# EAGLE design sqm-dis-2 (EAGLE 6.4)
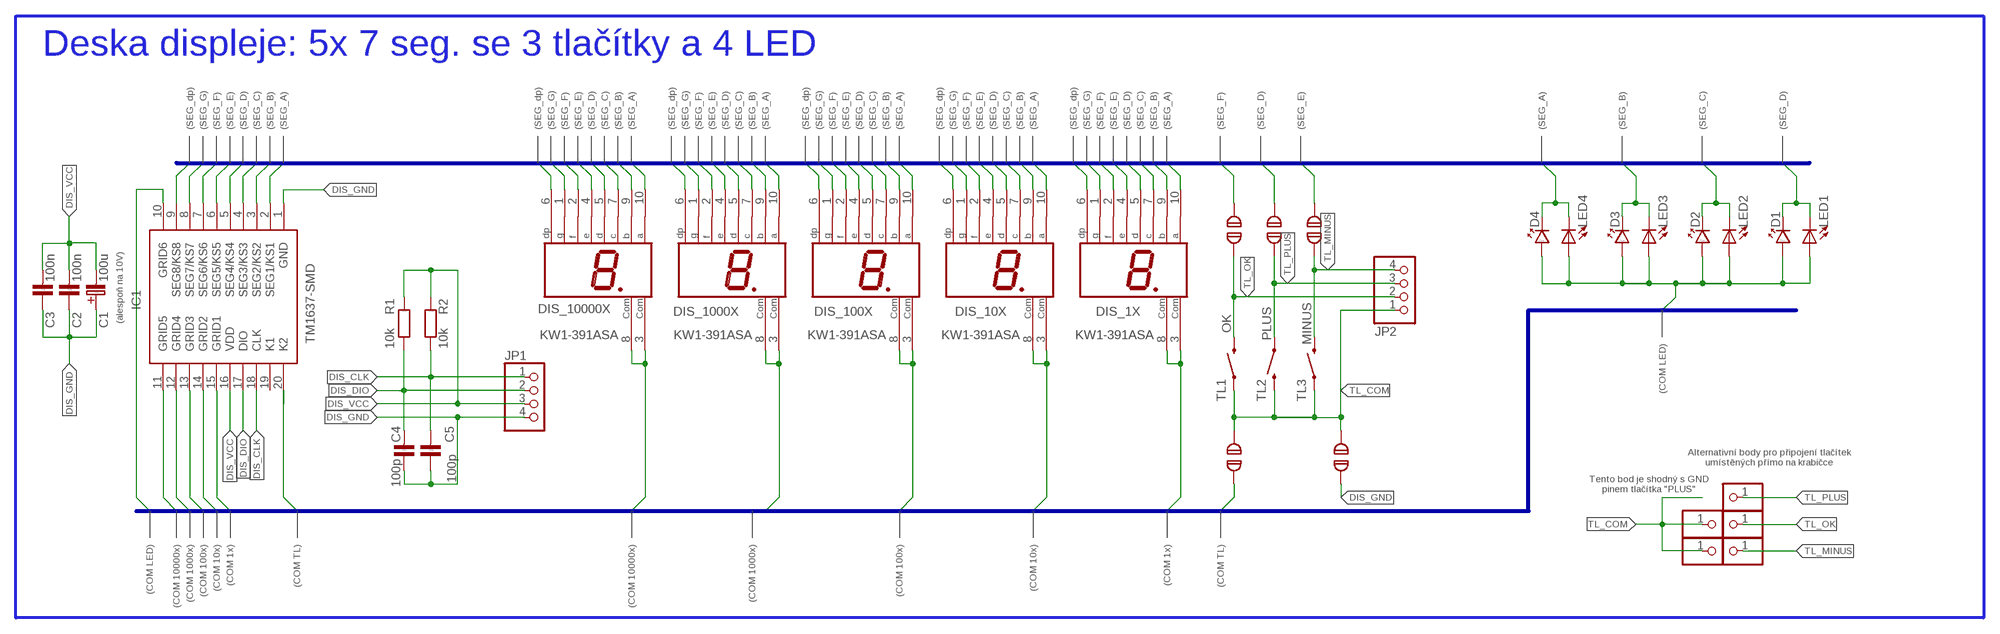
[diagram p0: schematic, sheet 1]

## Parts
C1  100u  C-ELEKTROLYT_2,5  [C-EL_2,5]
C2  100n  C-KERAMIK_SMD_0805  [0805]
C3  100n  C-KERAMIK_SMD_0805  [0805]
C4  100p  C-KERAMIK_SMD_0805  [0805]
C5  100p  C-KERAMIK_SMD_0805  [0805]
D1  LED_3  [LED_3]
D2  LED_3  [LED_3]
D3  LED_3  [LED_3]
D4  LED_3  [LED_3]
DIS_1X  KW1-391ASA  SC39-11SRWA  [HDSP-E]
DIS_10X  KW1-391ASA  SC39-11SRWA  [HDSP-E]
DIS_100X  KW1-391ASA  SC39-11SRWA  [HDSP-E]
DIS_1000X  KW1-391ASA  SC39-11SRWA  [HDSP-E]
DIS_10000X  KW1-391ASA  SC39-11SRWA  [HDSP-E]
IC1  TM1637-SMD  TM1637__SOP_  [SOIC127P1045X280-20N]
JP1  PINHD-1X4  [1X04]
JP2  PINHD-1X4  [1X04]
JP4  PINHD-1X1  [1X01]
JP5  PINHD-1X1  [1X01]
JP6  PINHD-1X1  [1X01]
JP7  PINHD-1X1  [1X01]
JP8  PINHD-1X1  [1X01]
LED1  LEDCHIP-LED0805  [CHIP-LED0805]
LED2  LEDCHIP-LED0805  [CHIP-LED0805]
LED3  LEDCHIP-LED0805  [CHIP-LED0805]
LED4  LEDCHIP-LED0805  [CHIP-LED0805]
R1  10k  R_SMD_0805  [0805]
R2  10k  R_SMD_0805  [0805]
SJ1  SJ  SOLDERJUMPER  [SJ_2S-NO]
SJ2  SJ  SOLDERJUMPER  [SJ_2S-NO]
SJ3  SJ  SOLDERJUMPER  [SJ_2S-NO]
SJ_COM  SJ  SOLDERJUMPER  [SJ_2S-NO]
SJ_GND  SJ  SOLDERJUMPER  [SJ_2S-NO]
TL1  OK  MOMENTARY-SWITCH-SPST-PTH-6.0MM  [TACTILE_SWITCH_PTH_6.0MM]
TL2  PLUS  MOMENTARY-SWITCH-SPST-PTH-6.0MM  [TACTILE_SWITCH_PTH_6.0MM]
TL3  MINUS  MOMENTARY-SWITCH-SPST-PTH-6.0MM  [TACTILE_SWITCH_PTH_6.0MM]

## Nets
COM_BUS0: DIS_1X.3(COM) DIS_1X.8(COM) IC1.15(GRID1)
COM_BUS1: DIS_10X.3(COM) DIS_10X.8(COM) IC1.14(GRID2)
COM_BUS2: DIS_100X.3(COM) DIS_100X.8(COM) IC1.13(GRID3)
COM_BUS3: DIS_1000X.3(COM) DIS_1000X.8(COM) IC1.12(GRID4)
COM_BUS4: DIS_10000X.3(COM) DIS_10000X.8(COM) IC1.11(GRID5)
COM_BUS5: IC1.20(K2) SJ_COM.1
COM_BUS6: D1.A D2.A D3.A D4.A IC1.10(GRID6) LED1.A LED2.A LED3.A LED4.A
DIS_CLK: C5.2 IC1.18(CLK) JP1.1 R2.1
DIS_DIO: C4.2 IC1.17(DIO) JP1.2 R1.1
DIS_GND: C1.C+(C_EL+) C2.1 C3.1 C4.1 C5.1 IC1.1(GND) JP1.4 SJ_GND.1
DIS_VCC: C1.C-(C_EL-) C2.2 C3.2 IC1.16(VDD) JP1.3 R1.2 R2.2
SEG_BUS0: D4.K DIS_1X.10(A) DIS_10X.10(A) DIS_100X.10(A) DIS_1000X.10(A) DIS_10000X.10(A) IC1.2(SEG1/KS1) LED4.C
SEG_BUS1: D3.K DIS_1X.9(B) DIS_10X.9(B) DIS_100X.9(B) DIS_1000X.9(B) DIS_10000X.9(B) IC1.3(SEG2/KS2) LED3.C
SEG_BUS2: D2.K DIS_1X.7(C) DIS_10X.7(C) DIS_100X.7(C) DIS_1000X.7(C) DIS_10000X.7(C) IC1.4(SEG3/KS3) LED2.C
SEG_BUS3: D1.K DIS_1X.5(D) DIS_10X.5(D) DIS_100X.5(D) DIS_1000X.5(D) DIS_10000X.5(D) IC1.5(SEG4/KS4) LED1.C SJ2.2
SEG_BUS4: DIS_1X.4(E) DIS_10X.4(E) DIS_100X.4(E) DIS_1000X.4(E) DIS_10000X.4(E) IC1.6(SEG5/KS5) SJ3.2
SEG_BUS5: DIS_1X.2(F) DIS_10X.2(F) DIS_100X.2(F) DIS_1000X.2(F) DIS_10000X.2(F) IC1.7(SEG6/KS6) SJ1.2
SEG_BUS6: DIS_1X.1(G) DIS_10X.1(G) DIS_100X.1(G) DIS_1000X.1(G) DIS_10000X.1(G) IC1.8(SEG7/KS7)
SEG_BUS7: DIS_1X.6(DP) DIS_10X.6(DP) DIS_100X.6(DP) DIS_1000X.6(DP) DIS_10000X.6(DP) IC1.9(SEG8/KS8)
TL_COM: JP2.1 JP7.1 JP8.1 SJ_COM.2 SJ_GND.2 TL1.1 TL2.3 TL3.1
TL_MINUS: JP2.4 JP6.1 SJ3.1 TL3.3
TL_OK: JP2.2 JP4.1 SJ1.1 TL1.3
TL_PLUS: JP2.3 JP5.1 SJ2.1 TL2.1
Unconnected: IC1.19(K1)

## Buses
SEG_BUS[0..7]
COM_BUS[0..6]

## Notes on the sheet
- Deska displeje: 5x 7 seg. se 3 tlačítky a 4 LED
- (SEG_dp) | (SEG_G) | (SEG_F) | (SEG_E) | (SEG_D) | (SEG_C) | (SEG_B) | (SEG_A) | (SEG_dp) | (SEG_G) | (SEG_F) | (SEG_E) | (SEG_D) | (SEG_C) | (SEG_B) | (SEG_A) | (SEG_dp) | (SEG_G) | (SEG_F) | (SEG_E) | (SEG_D) | (SEG_C) | (SEG_B) | (SEG_A) | (SEG_dp) | (SEG_G) | (SEG_F) | (SEG_E) | (SEG_D) | (SEG_C) | (SEG_B) | (SEG_A) | (SEG_dp) | (SEG_G) | (SEG_F) | (SEG_E) | (SEG_D) | (SEG_C) | (SEG_B) | (SEG_A) | (SEG_dp) | (SEG_G) | (SEG_F) | (SEG_E) | (SEG_D) | (SEG_C) | (SEG_B) | (SEG_A) | (SEG_F) | (SEG_D) | (SEG_E) | (SEG_A) | (SEG_B) | (SEG_C) | (SEG_D)
- (alespoň na 10V)
- (COM LED)
- Alternativní body pro připojení tlačítek
  umístěných přímo na krabičce
- Tento bod je shodný s GND
  pinem tlačítka "PLUS"
- (COM LED) | (COM 10000x) | (COM 1000x) | (COM 100x) | (COM 10x) | (COM 1x) | (COM TL) | (COM 10000x) | (COM 1000x) | (COM 100x) | (COM 10x) | (COM 1x) | (COM TL)

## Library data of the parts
C1 = #PaJa_30:C-ELEKTROLYT: Kondenzator - elektrolyticky
C2-C5 = #PaJa_30:C-KERAMIK: Kondenzator - keramicky
D1-D4 = #PaJa_30:LED: LED - jednobarevna
DIS_1X DIS_10X DIS_100X DIS_1000X DIS_10000X = display-hp:SC39-11SRWA: SINGLE DIGIT NUMERIC DISPLAY 9.9mm (0.39INCH) Source: SC39-11SRWA.pdf; OC_FARNELL: unknown; OC_NEWARK: unknown
IC1 = TM1637__SOP_:TM1637__SOP_: LED Drive Control Special Circuit Source: Datasheet; DESCRIPTION: LED Drive Control Special Circuit; HEIGHT: 2.8mm; MANUFACTURER_NAME: TITAN MICRO ELECTRONICS; MANUFACTURER_PART_NUMBER: TM1637 (SOP)
JP1 JP2 = pinhead:PINHD-1X4: PIN HEADER
JP4-JP8 = pinhead:PINHD-1X1: PIN HEADER
LED1-LED4 = adafruit:LED: LED
R1 R2 = #PaJa_30:R: Rezistor
SJ1-SJ3 SJ_COM SJ_GND = solderjump:SOLDERJUMPER: Pájecí propojka
TL1-TL3 = SparkFun-Switches:MOMENTARY-SWITCH-SPST: Momentary Switch (Pushbutton) - SPST; PROD_ID: SWCH-08441; SF_SKU: COM-00097

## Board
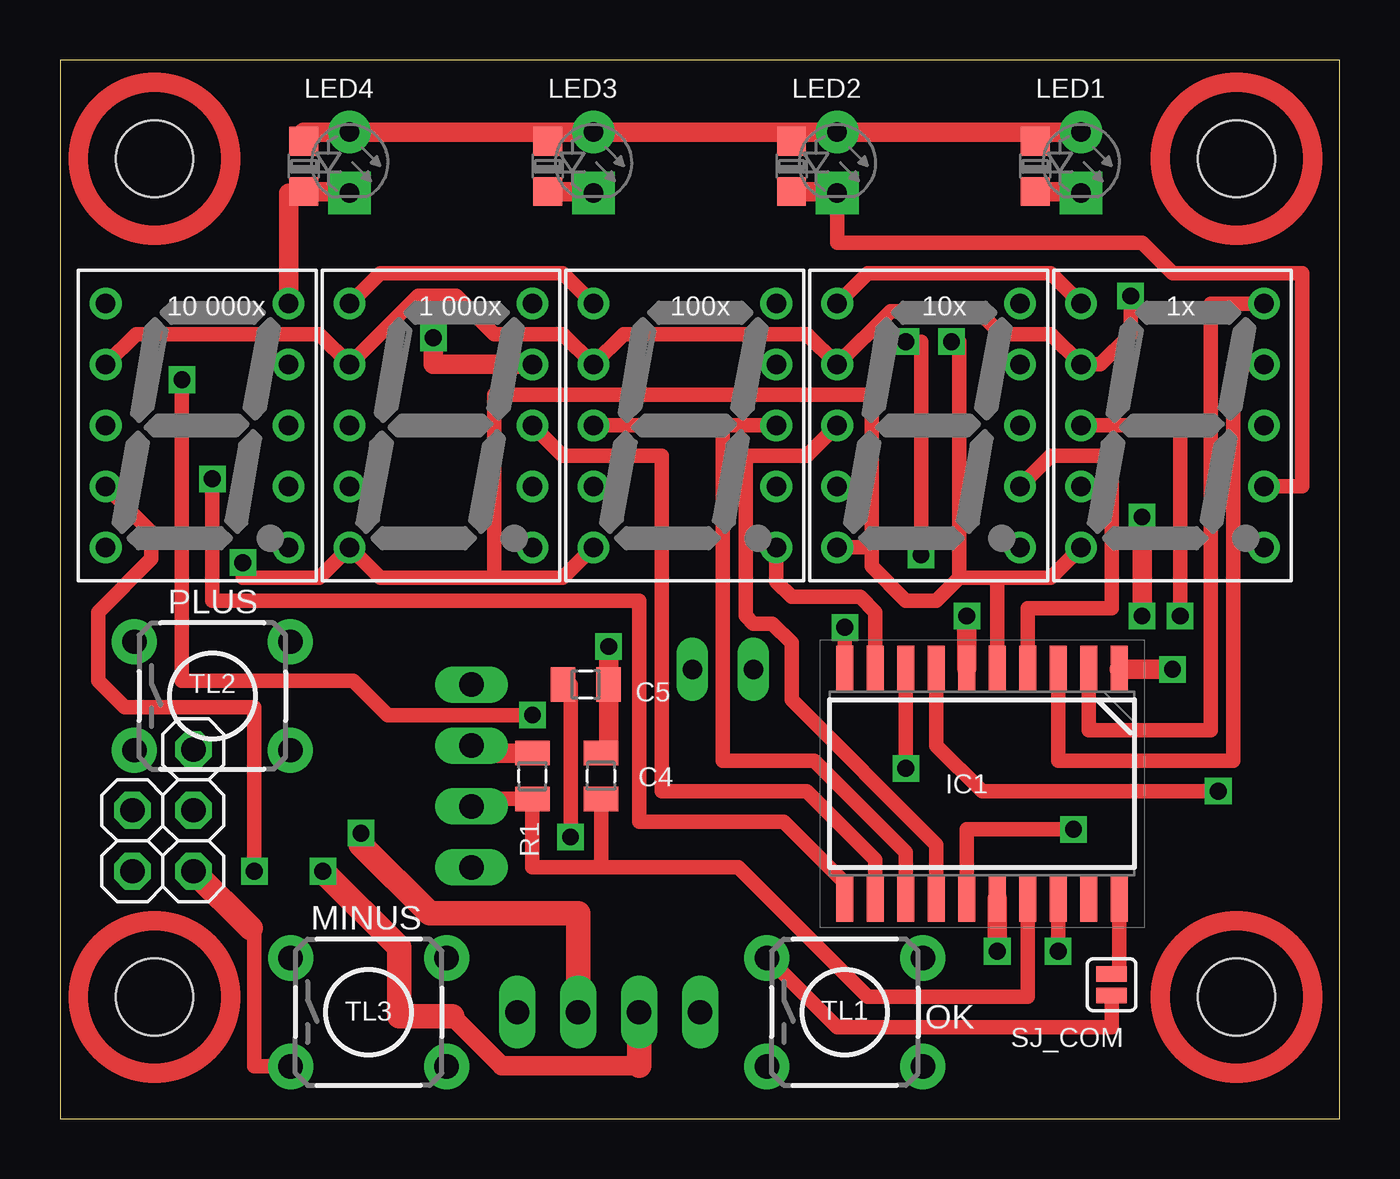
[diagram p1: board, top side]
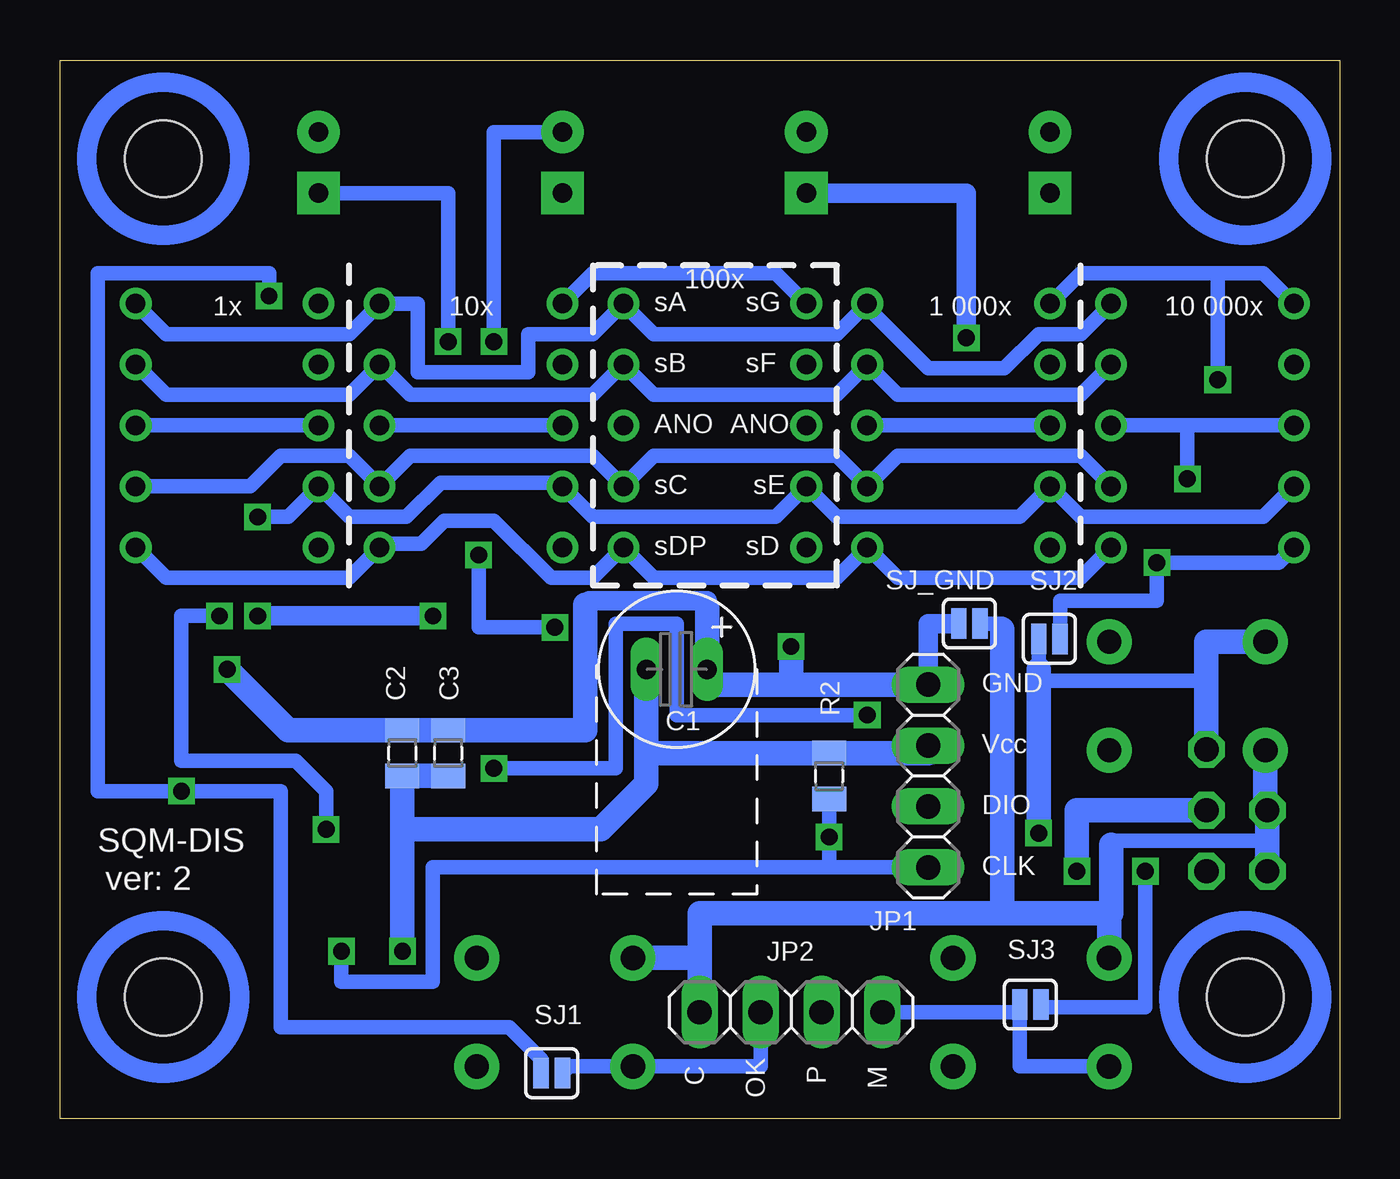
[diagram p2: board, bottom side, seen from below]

Size 53.32 x 44.12 mm. Coordinates in mm from the lower left corner, seen from the top.
Outline: 0,0 53.32,0 53.32,44.12 0,44.12 0,0
Copper layers (1*16): Top 0.035mm / dielectric 1.5mm / Bottom 0.035mm
Design rules "default *": minimum track width 10mil, minimum drill 24mil, track to track 8mil, track to pad 8mil, pad to pad 8mil, via to via 8mil, smd to smd 8mil, copper to edge 40mil, drill to drill 8mil, minimum pad ring 10mil, minimum via ring 8mil, stop-mask expansion 4mil, vias tented up to drill 0mil, thermal gap 10mil
Holes 3.2 mm at 49.02,5.08 3.94,40.01 49.02,40.01 3.94,5.08

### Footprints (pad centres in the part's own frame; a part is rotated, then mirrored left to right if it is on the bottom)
C-EL_2,5 = drill 0.813 pad 1.27 long: C+ -1.27,0; C- 1.27,0
0805 = smd 1.016 x 1.422: 1 -0.953,0; 2 0.953,0
LED_3 = drill 0.813 pad 1.778: A -1.27,0 | drill 0.813 pad 1.778 square: K 1.27,0
HDSP-E = drill 0.813: 1 -3.81,5.08; 2 -3.81,2.54; 3 -3.81,0; 4 -3.81,-2.54; 5 -3.81,-5.08; 6 3.81,-5.08; 7 3.81,-2.54; 8 3.81,0; 9 3.81,2.54; 10 3.81,5.08
SOIC127P1045X280-20N = smd 1.9 x 0.7: 1 -4.8,5.715; 2 -4.8,4.445; 3 -4.8,3.175; 4 -4.8,1.905; 5 -4.8,0.635; 6 -4.8,-0.635; 7 -4.8,-1.905; 8 -4.8,-3.175; 9 -4.8,-4.445; 10 -4.8,-5.715; 11 4.8,-5.715; 12 4.8,-4.445; 13 4.8,-3.175; 14 4.8,-1.905; 15 4.8,-0.635; 16 4.8,0.635; 17 4.8,1.905; 18 4.8,3.175; 19 4.8,4.445; 20 4.8,5.715
1X04 = drill 1.016 long: 1 -3.81,0; 2 -1.27,0; 3 1.27,0; 4 3.81,0
1X01 = drill 1.016 octagon: 1 0,0
CHIP-LED0805 = smd 1.2 x 1.2: A 0,-1.05; C 0,1.05
SJ_2S-NO = smd 0.635 x 1.27: 1 0,0; 2 0.889,0
TACTILE_SWITCH_PTH_6.0MM = drill 1.016 pad 1.88: 1 -3.251,2.261; 2 3.251,2.261; 3 -3.251,-2.261; 4 3.251,-2.261

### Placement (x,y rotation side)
C1  27.62,18.73 180 bottom
C2  39.05,15.24 270 bottom
C3  37.15,15.24 270 bottom
C4  22.54,14.29 270 top
C5  21.91,18.1 180 top
D1  42.55,39.85 270 top
D2  32.38,39.85 270 top
D3  22.23,39.85 270 top
D4  12.06,39.85 270 top
DIS_1X  46.35,28.89 0 top
DIS_10X  36.2,28.89 0 top
DIS_100X  26.04,28.89 0 top
DIS_1000X  15.88,28.89 0 top
DIS_10000X  5.71,28.89 0 top
IC1  38.42,13.97 270 top
JP1  17.14,14.29 90 bottom
JP2  22.86,4.45 0 bottom
JP4  5.56,12.86 0 top
JP5  5.56,15.4 0 top
JP6  5.56,10.32 0 top
JP7  3.02,12.86 0 top
JP8  3.02,10.32 0 top
LED1  40.64,39.69 180 top
LED2  30.48,39.69 180 top
LED3  20.32,39.69 180 top
LED4  10.16,39.69 180 top
R1  19.68,14.29 90 top
R2  21.27,14.29 90 bottom
SJ1  32.38,1.91 180 bottom
SJ2  12.54,20 0 bottom
SJ3  13.34,4.76 0 bottom
SJ_COM  43.81,6.03 270 top
SJ_GND  15.88,20.64 0 bottom
TL1  32.7,4.45 0 top
TL2  6.35,17.62 0 top
TL3  12.86,4.45 0 top

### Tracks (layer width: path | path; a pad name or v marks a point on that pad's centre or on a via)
COM_BUS0  (via drill 0.7)
  Top 0.61: DIS_1X.3 46.67,28.89 v46.67,20.95 | v42.23,12.06 37.78,12.06 IC1.15
  Bottom 0.61: v46.67,20.95 48.26,20.95 48.26,14.92 43.5,14.92 42.23,13.65 v42.23,12.06 | DIS_1X.8 DIS_1X.3
COM_BUS1
  Top 0.61: DIS_10X.3 31.11,27.62 28.57,27.62 28.57,20.95 28.89,20.64 29.69,20.64 30.48,19.84 30.48,17.46 36.51,11.43 IC1.14
  Bottom 0.61: DIS_10X.3 DIS_10X.8
COM_BUS2
  Top 0.61: 27.62,28.89 27.62,14.92 31.43,14.92 35.24,11.11 IC1.13 | 27.62,28.89 DIS_100X.3 | 27.62,28.89 DIS_100X.8
COM_BUS3
  Top 0.61: DIS_1000X.8 20.95,27.62 25.08,27.62 25.08,13.65 31.11,13.65 33.97,10.79 IC1.12
  Bottom 0.61: DIS_1000X.3 DIS_1000X.8
COM_BUS4  (via drill 0.7)
  Top 0.61: v6.35,26.67 6.35,21.59 24.13,21.59 24.13,12.38 30.16,12.38 32.7,9.84 IC1.11
  Bottom 0.61: DIS_10000X.3 6.35,28.89 | 6.35,28.89 v6.35,26.67 | DIS_10000X.8 6.35,28.89
COM_BUS5
  Top 0.61: IC1.20 44.13,6.03 SJ_COM.1
COM_BUS6  (via drill 0.7)
  Top 0.61: IC1.10 v32.7,20.48 | v35.88,23.5 35.88,32.38 v35.24,32.38
  Top 0.813: D2.A D3.A 20.32,41.12 | D2.A D1.A 40.64,41.12 LED1.A | D2.A 30.48,41.12 LED2.A | 20.32,41.12 D4.A 10.16,41.12 LED4.A | 20.32,41.12 LED3.A
  Bottom 0.61: v32.7,20.48 35.88,20.48 v35.88,23.5 | v35.24,32.38 35.24,41.12 D2.A
DIS_CLK  (via drill 0.7)
  Top 0.61: IC1.18 v41.59,6.99 | C5.2 21.27,18.1 v21.27,11.75
  Bottom 0.61: v41.59,6.99 41.59,5.71 37.78,5.71 37.78,10.48 21.27,10.48 | JP1.1 21.27,10.48 | R2.1 v21.27,11.75 21.27,10.48
DIS_DIO
  Top 0.61: IC1.17 40.32,5.08 33.66,5.08 28.26,10.48 22.54,10.48 | JP1.2 17.14,13.34 R1.1 19.68,10.48 22.54,10.48 | C4.2 22.54,10.48
DIS_GND  (via drill 0.7)
  Top 0.61: IC1.1 44.13,18.73
  Top 0.813: 44.13,18.73 v46.35,18.73 | v22.86,19.68 C5.1 22.86,15.24 C4.1
  Bottom 0.61: SJ_GND.1 16.03,20.64
  Bottom 0.813: 31.43,21.43 31.27,21.59 26.35,21.59 26.35,21.27 | 16.03,20.64 17.14,20.64 JP1.4
  Bottom 1.016: JP1.4 C5.1 | v22.86,19.68 C5.1 | C5.1 26.35,18.1 C1.C+ 26.35,21.27 | 31.43,21.43 31.43,16.19 C3.1 C2.1 43.81,16.19 v46.35,18.73
DIS_VCC  (via drill 0.7)
  Top 0.813: IC1.16 v39.05,6.99 | JP1.3 17.14,15.24 R1.2
  Bottom 1.016: v39.05,6.99 39.05,12.06 | 39.05,12.06 C2.2 C3.2 | 28.89,15.24 C1.C- | 28.89,15.24 R2.2 17.14,15.24 JP1.3 | 28.89,15.24 28.89,13.97 30.8,12.06 39.05,12.06
SEG_BUS0
  Top 0.61: IC1.2 42.86,16.19 47.94,16.19 47.94,33.97 DIS_1X.10
  Top 0.813: D4.K 12.06,38.64 LED4.C 10.16,38.58 9.53,38.58 DIS_10000X.10
  Bottom 0.61: DIS_1X.10 48.9,32.7 41.27,32.7 DIS_10X.10 38.42,33.97 38.42,31.11 33.81,31.11 33.81,32.7 31.11,32.7 DIS_100X.10 28.57,32.7 20.95,32.7 DIS_1000X.10 19.68,33.81 17.14,31.27 13.97,31.27 12.54,32.7 10.79,32.7 DIS_10000X.10
SEG_BUS1  (via drill 0.7)
  Top 0.61: IC1.3 41.59,14.92 48.9,14.92 48.9,31.43 DIS_1X.9
  Top 0.813: LED3.C 22.23,38.64 D3.K | DIS_1000X.9 15.56,31.43 v15.56,32.54
  Bottom 0.61: DIS_10000X.9 10.79,30.16 18.41,30.16 DIS_1000X.9 20.95,30.16 28.57,30.16 DIS_100X.9 31.11,30.16 38.73,30.16 DIS_10X.9 41.27,30.16 48.9,30.16 DIS_1X.9
  Bottom 0.813: v15.56,32.54 15.56,38.58 D3.K
SEG_BUS2
  Top 0.61: IC1.4 40.32,21.27 43.81,21.27 43.81,27.62 41.27,27.62 DIS_10X.7 | D2.K 32.38,36.51 45.09,36.51 46.35,35.24 51.75,35.24 51.75,26.35 DIS_1X.7
  Top 0.813: LED2.C 32.38,38.64 D2.K
  Bottom 0.61: DIS_10000X.7 10.79,27.62 18.41,27.62 DIS_1000X.7 20.95,27.62 28.57,27.62 DIS_100X.7 31.11,27.62 38.73,27.62 DIS_10X.7 41.27,27.62 44.13,27.62 45.4,26.35 DIS_1X.7
SEG_BUS3  (via drill 0.7)
  Top 0.61: 18.1,22.54 13.34,22.54 DIS_1000X.5 10.79,22.54 7.62,22.54 v7.62,23.18 | DIS_100X.5 20.95,22.54 18.1,22.54 | DIS_10X.5 33.81,23.81 | 37.47,22.54 36.51,21.59 35.24,21.59 33.81,23.02 33.81,23.81 | 37.47,22.54 39.05,22.54 | 39.05,22.54 41.27,22.54 DIS_1X.5 41.59,22.86 | 18.1,22.54 18.1,30.16 33.81,30.16 33.81,23.81 | IC1.5 39.05,22.54 | 37.47,22.54 37.47,32.38 v37.15,32.38
  Top 0.813: LED1.C 42.55,38.64 D1.K
  Bottom 0.61: DIS_10000X.5 2.54,23.18 v7.62,23.18 7.62,21.59 11.65,21.59 SJ2.2 | v37.15,32.38 37.15,38.58 D1.K
SEG_BUS4  (via drill 0.7)
  Top 0.61: DIS_10000X.4 3.81,24.45 3.81,23.34 1.59,21.11 1.59,18.26 2.7,17.14 8.1,17.14 v8.1,10.32
  Top 0.813: IC1.6 v37.78,20.95 | v45.09,20.95 v45.09,25.08
  Bottom 0.61: DIS_10000X.4 3.17,25.08 10.79,25.08 DIS_1000X.4 13.34,25.08 20.95,25.08 DIS_100X.4 23.5,25.08 31.11,25.08 DIS_10X.4 32.38,26.51 37.47,26.51 38.89,25.08 41.27,25.08 DIS_1X.4 43.81,25.08 v45.09,25.08 | SJ3.2 12.45,4.65 8.1,4.65 v8.1,10.32
  Bottom 0.813: v37.78,20.95 v45.09,20.95
SEG_BUS5  (via drill 0.7)
  Top 0.61: DIS_10000X.2 3.17,32.7 10.79,32.7 DIS_1000X.2 14.92,34.29 16.51,34.29 18.1,32.7 20.95,32.7 DIS_100X.2 23.5,32.7 31.11,32.7 DIS_10X.2 34.61,33.66 38.26,33.66 39.21,32.7 41.27,32.7 DIS_1X.2 43.34,31.43 44.61,32.7 v44.61,34.29 | v48.26,13.65 38.42,13.65 36.51,15.56 IC1.7
  Bottom 0.61: v44.61,34.29 44.61,35.24 51.75,35.24 51.75,13.65 v48.26,13.65 44.13,13.65 44.13,3.81 34.61,3.81 33.27,2.48 SJ1.2
SEG_BUS6  (via drill 0.7)
  Top 0.61: DIS_1X.1 41.27,35.24 33.66,35.24 DIS_10X.1 | DIS_1000X.1 13.34,35.24 20.95,35.24 DIS_100X.1 | IC1.8 v35.24,14.61 | v5.08,30.8 5.08,18.26 12.22,18.26 13.65,16.83 v19.68,16.83
  Bottom 0.61: DIS_10000X.1 3.17,35.24 5.08,35.24 | 5.08,35.24 10.79,35.24 DIS_1000X.1 | DIS_10X.1 31.11,35.24 23.5,35.24 DIS_100X.1 | v35.24,14.61 30.16,14.61 30.16,20.64 27.62,20.64 27.62,16.83 v19.68,16.83 | v5.08,30.8 5.08,35.24
SEG_BUS7
  Top 0.61: IC1.9 33.97,21.11 33.34,21.75 30.48,21.75 29.84,22.38 DIS_100X.6
  Bottom 0.61: DIS_10000X.6 10.79,22.54 18.41,22.54 DIS_1000X.6 20.95,22.54 28.57,22.54 DIS_100X.6 31.11,22.54 32.86,22.54 35.24,24.92 37.31,24.92 38.26,23.97 39.85,23.97 DIS_10X.6 41.27,22.54 48.9,22.54 DIS_1X.6
TL_COM
  Top 0.61: TL1.1 29.49,6.71 32.38,3.81 43.81,3.81 SJ_COM.2
  Bottom 0.61: SJ_GND.2 14.05,20.64 14.05,20.4 | JP8.1 3.02,11.59 9.53,11.59 9.53,11.43
  Bottom 1.016: 9.6,8.57 TL3.1 | JP2.1 26.67,6.71 | 14.05,8.57 26.67,8.57 26.67,6.71 | 14.05,8.57 9.6,8.57 | 9.6,8.57 9.53,8.57 9.53,11.43 | 26.67,6.71 TL1.1 | TL2.3 3.1,12.86 JP7.1 JP8.1 | 14.05,20.4 14.05,8.57
TL_MINUS
  Top 0.61: 7.94,7.94 8.1,7.94 8.1,2.18 TL3.3
  Top 1.016: JP6.1 7.94,7.94
  Bottom 0.61: TL3.3 13.34,2.18 13.34,4.45 | 13.34,4.45 SJ3.1 | JP2.4 13.34,4.45
TL_OK  (via drill 0.7)
  Top 0.813: 16.35,4.29 18.41,2.22 24.13,2.22
  Top 1.016: 24.13,2.22 JP2.2 | v10.95,10.32 14.13,7.14 14.13,4.29 16.35,4.29
  Bottom 0.61: SJ1.1 32.11,2.18 TL1.3 24.13,2.18 JP2.2
  Bottom 1.016: JP4.1 10.95,12.86 v10.95,10.32
TL_PLUS  (via drill 0.7)
  Top 1.016: JP2.3 21.59,8.57 15.4,8.57 12.54,11.43 v12.54,11.91
  Bottom 0.61: JP5.1 5.56,18.26 12.54,18.26 12.54,18.73 SJ2.1
  Bottom 1.016: TL2.1 5.56,19.88 JP5.1 | 12.54,18.73 v12.54,11.91
(copper drawn outside any net)
  shapes: Bottom circle x4, Top circle x4

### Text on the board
tPlace: 10 000x | 1 000x | 100x | 10x | 1x | PLUS | MINUS | OK
bPlace: 100x | 10 000x | 1 000x | sG | sA | 10x | 1x | sF | sB | ANO | ANO | sE | sC | sD | sDP | GND | Vcc | DIO | SQM-DIS | CLK | ver: 2 | OK | M | P | C
tDocu: tl_PLUS | tl_OK | tl_MINUS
